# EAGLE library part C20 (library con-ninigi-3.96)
NINIGI
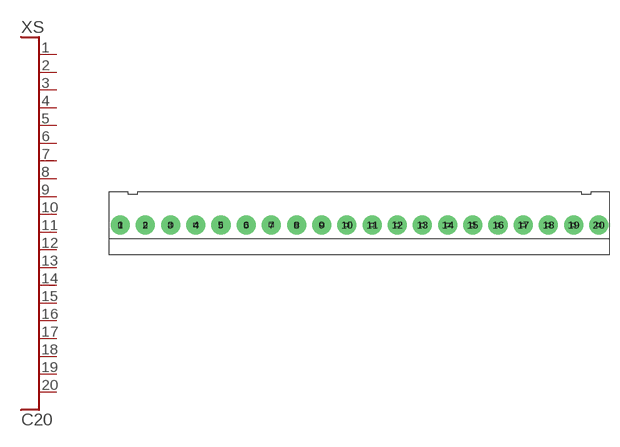
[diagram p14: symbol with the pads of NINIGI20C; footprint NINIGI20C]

Designator prefix XS

## C20  [NINIGI20C]
1  P$1
2  P$2
3  P$3
4  P$4
5  P$5
6  P$6
7  P$7
8  P$8
9  P$9
10  P$10
11  P$11
12  P$12
13  P$13
14  P$14
15  P$15
16  P$16
17  P$17
18  P$18
19  P$19
20  P$20

## Footprint NINIGI20C (pad centres in mm)
drill 1.6 pad 3: 1 -37.62,0; 2 -33.66,0; 3 -29.7,0; 4 -25.74,0; 5 -21.78,0; 6 -17.82,0; 7 -13.86,0; 8 -9.9,0; 9 -5.94,0; 10 -1.98,0; 11 1.98,0; 12 5.94,0; 13 9.9,0; 14 13.86,0; 15 17.82,0; 16 21.78,0; 17 25.74,0; 18 29.7,0; 19 33.66,0; 20 37.62,0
